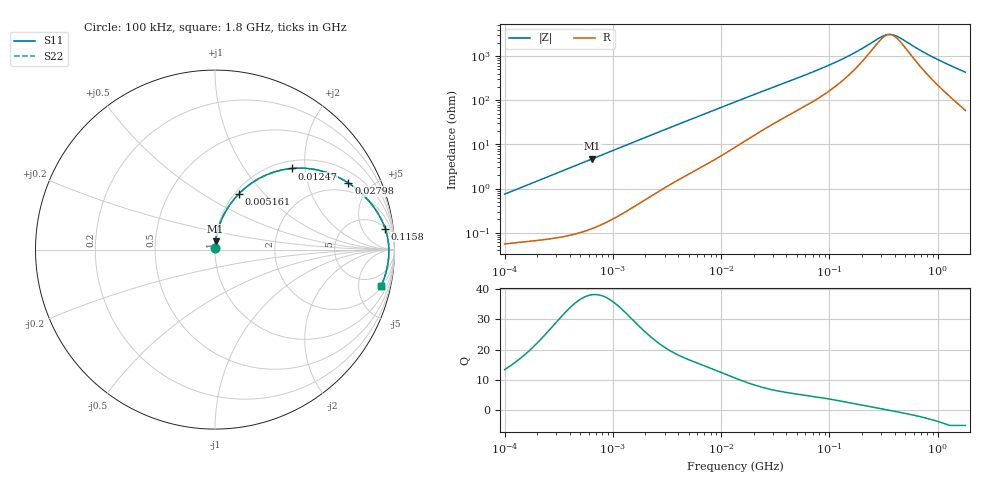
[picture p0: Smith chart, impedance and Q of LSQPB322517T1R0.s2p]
! LSQPB322517T1R0  S-PARAMETER MODEL  ( General Type )
! Model Generated by TAIYO YUDEN Corporation (http://www.ty-top.com)
! Version 2.0
! TAIYO YUDEN Control No. 100810NC14SB-FKC
! Copyright(c) 2008 TAIYO YUDEN CO.,LTD. All Rights Reserved.
! Product Description (link to TY-COMPAS)
! https://ds.yuden.co.jp/TYCOMPAS/or/detail?pn=LSQPB322517T1R0M&u=M
! Products Name : Inductors
! Characteristics :
!  Inductance : 1.0 uH , SRF(min) : 220 MHz , DC Resistance(max) : 0.0516 Ohm
!  Rated Current : Saturation :2400 mA , Temp Rise : 2200 mA (40 degC)
!  Case Size : 3.2 x 2.5 / 0.126 x 0.098 [mm/inch] , Thickness : 1.7 / 0.068 [mm/inch]
!  (Conditions: Temperature = 25 degC , DC Bias Current/Voltage = 0A / 0V)
! External Node Assignments :
!  1  o---GGG---o  2
! GND o---------o GND
! Frequency Range : 0.1MHz  -  1800MHz  [ 402 STEP ]
# MHz S RI R 50
! Freq[MHz].  S11 Real  S11 Imag  S21 Real  S21 Imag  S12 Real  S12 Imag  S22 Real  S22 Imag
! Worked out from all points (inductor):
!   401 points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, 100 kHz to 1.8 GHz, reference 50 ohm
!   read as one part in series: L = 1.18 uH near 105 kHz
!   highest Q = 38.2 at 643.4 kHz (marker M1), where L = 1.16 uH
!   self-resonance near 358.3 MHz
!   S11 on the Smith chart (normalised r, x): 100 kHz: 1.00, +0.01; 5.161 MHz: 1.04, +0.73; 12.47 MHz: 1.15, +1.70; 27.98 MHz: 1.52, +3.65; 115.8 MHz: 5, +14; 1.8 GHz: 2.18, -8.61
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0.1  0.000608 0.00742  0.9994 -0.00742  0.9994 -0.00742  0.000608 0.00742
0.516129  0.00244 0.0377  0.9976 -0.0377  0.9976 -0.0377  0.00244 0.0377
0.643431  0.00343 0.0469  0.9966 -0.0469  0.9966 -0.0469  0.00343 0.0469
1.374945  0.013 0.0985  0.987 -0.0985  0.987 -0.0985  0.013 0.0985
2.66389  0.0431 0.1817  0.9569 -0.1817  0.9569 -0.1817  0.0431 0.1817
5.161158  0.1315 0.309  0.8685 -0.309  0.8685 -0.309  0.1315 0.309
7.827017  0.2445 0.3956  0.7555 -0.3956  0.7555 -0.3956  0.2445 0.3956
12.46584  0.429 0.452  0.571 -0.452  0.571 -0.452  0.429 0.452
13.41641  0.4612 0.4538  0.5388 -0.4538  0.5388 -0.4538  0.4612 0.4538
18.44729  0.5973 0.4371  0.4027 -0.4371  0.4027 -0.4371  0.5973 0.4371
27.97575  0.7433 0.371  0.2567 -0.371  0.2567 -0.371  0.7433 0.371
42.42587  0.8422 0.2877  0.1578 -0.2877  0.1578 -0.2877  0.8422 0.2877
69.24595  0.9115 0.196  0.0885 -0.196  0.0885 -0.196  0.9115 0.196
115.8234  0.9481 0.1173  0.0519 -0.1173  0.0519 -0.1173  0.9481 0.1173
180.0045  0.9622 0.0649  0.0378 -0.0649  0.0378 -0.0649  0.9622 0.0649
301.0823  0.9683 0.0155  0.0317 -0.0155  0.0317 -0.0155  0.9683 0.0155
357.3983  0.9689 0.00022  0.0311 -0.00022  0.0311 -0.00022  0.9689 0.00022
384.6512  0.9689 -0.0063  0.0311 0.0063  0.0311 0.0063  0.9689 -0.0063
424.248  0.9689 -0.015  0.0311 0.015  0.0311 0.015  0.9689 -0.015
863.2311  0.9615 -0.0879  0.0385 0.0879  0.0385 0.0879  0.9615 -0.0879
1277.433  0.9481 -0.1427  0.0519 0.1427  0.0519 0.1427  0.9481 -0.1427
1800  0.9244 -0.2044  0.0756 0.2044  0.0756 0.2044  0.9244 -0.2044
